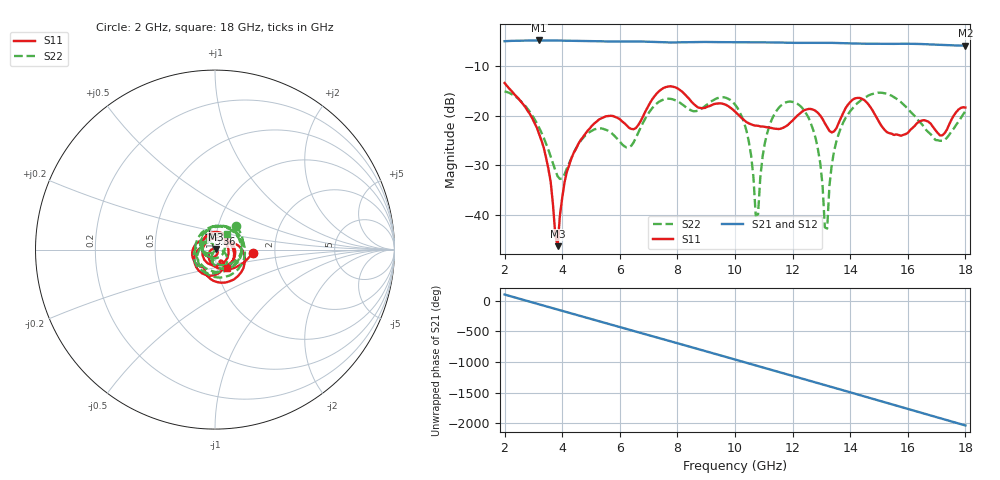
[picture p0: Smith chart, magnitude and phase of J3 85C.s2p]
!Agilent Technologies,E8363B,SG43030131,A.07.50.48
!Agilent E8363B: A.07.50.48
!Date: Wednesday, December 17, 2025 22:40:55
!Correction: S11(Full 2 Port(1,2))
!S21(Full 2 Port(1,2))
!S12(Full 2 Port(1,2))
!S22(Full 2 Port(1,2))
!S2P File: Measurements: S11, S21, S12, S22:
# Hz S  dB  R 50
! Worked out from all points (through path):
!   201 points, 2 GHz to 18 GHz, reference 50 ohm
!   highest |S21| = -4.92 dB at 3.2 GHz (marker M1); lowest = -6.0 dB at 18 GHz (marker M2)
!   group delay of S21, straight-line fit = 371 ps
!   lowest |S11| = -46.2 dB at 3.84 GHz (marker M3), VSWR 1.01, Z = 50.3 + j0.345 ohm
!   |S11| at or under -10 dB: start of sweep to end of sweep
!   |S22| runs from -42.7 to -15.2 dB; largest |S21 - S12| = 0.0025
!   S11 on the Smith chart (normalised r, x): 2 GHz: 1.54, -0.05; 5.36 GHz: 0.92, +0.16; 18 GHz: 1.12, -0.23
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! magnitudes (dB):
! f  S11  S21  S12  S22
! 2 GHz  -13.5  -5.1  -5.1  -15.2
! 3.2 GHz  -23.7  -4.9  -4.9  -22.4
! 3.6 GHz  -33.3  -4.9  -4.9  -28.2
! 3.84 GHz  -46.2  -4.9  -4.9  -32.2
! 4.16 GHz  -31.3  -5.0  -5.0  -30.6
! 4.72 GHz  -24.3  -5.0  -5.0  -24.5
! 5.36 GHz  -20.6  -5.1  -5.1  -22.6
! 6.32 GHz  -22.4  -5.1  -5.1  -26.3
! 7.36 GHz  -15.1  -5.3  -5.3  -17.2
! 10 GHz  -19.2  -5.3  -5.3  -17.8
! 10.48 GHz  -21.6  -5.3  -5.3  -25.2
! 10.72 GHz  -22.0  -5.3  -5.3  -40.1
! 11.04 GHz  -22.3  -5.3  -5.3  -25.4
! 11.44 GHz  -22.7  -5.3  -5.3  -19.0
! 12.72 GHz  -18.8  -5.4  -5.4  -23.0
! 13.2 GHz  -22.3  -5.4  -5.4  -42.7
! 13.36 GHz  -23.4  -5.4  -5.4  -29.9
! 13.76 GHz  -19.5  -5.5  -5.5  -21.3
! 14.4 GHz  -16.6  -5.6  -5.6  -16.8
! 15.36 GHz  -23.5  -5.6  -5.6  -15.8
! 16.96 GHz  -22.9  -5.8  -5.8  -24.9
! 18 GHz  -18.4  -6.0  -6.0  -19.1
